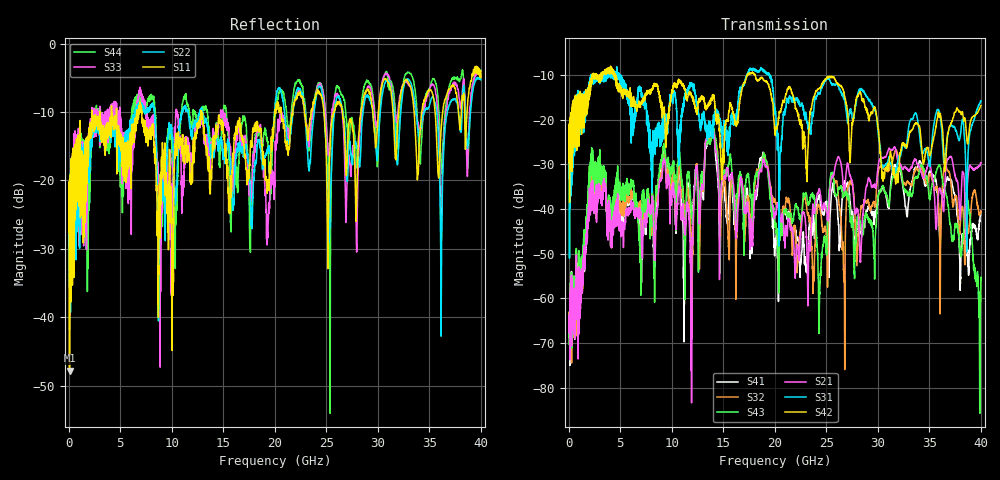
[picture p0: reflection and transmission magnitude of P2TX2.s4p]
!Agilent Technologies,N5245A,MY49151084,A.09.20.08
!Agilent N5245A: A.09.20.08
!Date: Thursday, March 01, 2012 11:51:38
!Correction: S11(Full 4 Port(1,2,3,4))
!S12(Full 4 Port(1,2,3,4))
!S13(Full 4 Port(1,2,3,4))
!S14(Full 4 Port(1,2,3,4))
!S21(Full 4 Port(1,2,3,4))
!S22(Full 4 Port(1,2,3,4))
!S23(Full 4 Port(1,2,3,4))
!S24(Full 4 Port(1,2,3,4))
!S31(Full 4 Port(1,2,3,4))
!S32(Full 4 Port(1,2,3,4))
!S33(Full 4 Port(1,2,3,4))
!S34(Full 4 Port(1,2,3,4))
!S41(Full 4 Port(1,2,3,4))
!S42(Full 4 Port(1,2,3,4))
!S43(Full 4 Port(1,2,3,4))
!S44(Full 4 Port(1,2,3,4))
!S4P File: Measurements: <S11,S12,S13,S14>,
!<S21,S22,S23,S24>,
!<S31,S32,S33,S34>,
!<S41,S42,S43,S44>:
# Hz S  dB  R 50
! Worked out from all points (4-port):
!   3996 points, 50 MHz to 40 GHz, reference 50 ohm
!   strongest paths, dB at 50 MHz, 10.04 GHz, 20.03 GHz, 30.02 GHz, 40 GHz:
!     S42: -23.5, -13.5, -22.8, -21.8, -16.8
!     S31: -24.6, -14.7, -17.2, -22.2, -15.8
!     S21: -66.4, -36.5, -41.0, -30.7, -29.7
!     S43: -63.5, -31.2, -43.5, -37.1, -56.0
!     S32: -64.0, -33.8, -37.7, -31.7, -40.4
!     S41: -65.6, -33.8, -46.9, -37.8, -40.6
!   lowest |S11| = -47.8 dB at 90 MHz (marker M1), VSWR 1.01, Z = 50.2 + j0.375 ohm
!   |S11| at or under -10 dB: start of sweep to 2.239 GHz; 7.092 GHz to 12.84 GHz (5.75 GHz wide, 57.7 % of centre); 12.9 GHz to 19.99 GHz (7.09 GHz wide, 43.1 % of centre)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
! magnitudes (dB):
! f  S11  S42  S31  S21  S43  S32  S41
! 50 MHz  -21.8  -23.5  -24.6  -66.4  -63.5  -64.0  -65.6
! 90 MHz  -47.8  -38.5  -51.0  -67.2  -65.7  -66.7  -66.3
! 2.21 GHz  -12.3  -11.8  -11.7  -34.0  -27.7  -29.6  -31.9
! 11.89 GHz  -19.8  -14.2  -12.0  -76.1  -40.0  -49.6  -40.6
! 14.05 GHz  -14.6  -14.8  -19.6  -22.6  -21.5  -22.1  -22.9
! 23.29 GHz  -12.8  -22.3  -21.3  -50.9  -38.7  -41.4  -46.3
! 40 GHz  -5.0  -16.8  -15.8  -29.7  -56.0  -40.4  -40.6
